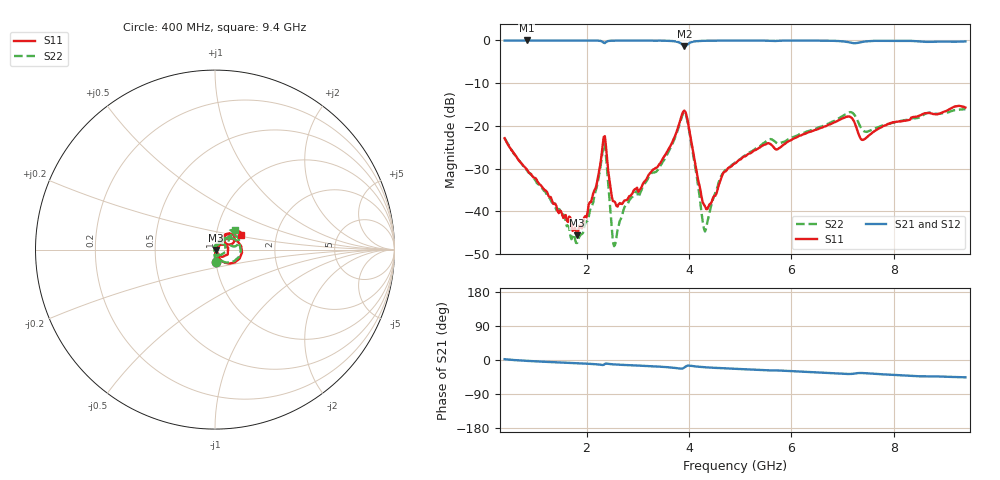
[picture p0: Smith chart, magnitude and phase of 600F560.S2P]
!  American Technical Ceramics  Date:  11/23/05
!  One Norden Lane
!  Huntington Station,  NY.  11746-2102
!  Tel:  (631) 622-4700  Fax:  (631) 622-4748
!  Part Number  600F560  Mounting Orientation: Horizontal
!  Description: Ultra Low ESR Microwave capacitors
!  Application: Coupling, Bypass, Tuning, DC Block
!  Filters, Matching
# GHZ S DB R 50
! Freq  |S11|  S11 Ph  |S21|  S21 Ph  |S12|  S12 Ph  |S22|  S22 Ph
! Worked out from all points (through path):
!   401 points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, 400 MHz to 9.4 GHz, reference 50 ohm
!   highest |S21| = 0.00 dB at 828 MHz (marker M1); lowest = -1.3 dB at 3.91 GHz (marker M2)
!   group delay of S21, straight-line fit = 14.1 ps
!   lowest |S11| = -45.6 dB at 1.818 GHz (marker M3), VSWR 1.01, Z = 50.5 - j0.172 ohm
!   |S11| at or under -10 dB: start of sweep to end of sweep
!   |S22| runs from -48.1 to -16.1 dB; largest |S21 - S12| = 0.0045
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0.4  -22.87 -86.8  -0.02 2.2  -0.03 2.2  -22.88 -87.6
0.828  -30.07 -87.9  0.00 -2.2  -0.02 -2.2  -30.23 -93.3
1.818  -45.56 -18.9  -0.01 -8.6  -0.02 -8.6  -47.37 179.0
1.908  -43.97 9.3  -0.01 -9.1  -0.02 -9.1  -45.29 137.7
2.178  -34.57 41.4  -0.02 -11.1  -0.04 -11.1  -35.20 95.1
2.335  -22.58 9.2  -0.54 -12.8  -0.55 -12.7  -24.12 25.2
2.38  -24.83 -45.1  -0.38 -9.5  -0.40 -9.4  -27.00 -42.0
2.515  -37.57 -34.1  -0.05 -11.4  -0.06 -11.4  -47.01 -140.2
2.56  -37.92 -24.2  -0.04 -11.8  -0.05 -11.8  -47.72 155.4
2.785  -37.34 19.0  -0.04 -13.4  -0.06 -13.3  -38.43 103.7
3.415  -29.06 54.0  -0.04 -17.5  -0.06 -17.5  -29.83 68.0
3.91  -16.40 -6.2  -1.33 -19.9  -1.34 -19.9  -16.82 -2.7
4  -20.48 -51.6  -0.68 -14.9  -0.70 -14.9  -20.80 -51.2
4.315  -38.84 -16.1  -0.08 -19.1  -0.09 -19.1  -44.70 -2.5
4.63  -32.25 62.7  -0.05 -21.4  -0.06 -21.4  -31.65 61.5
4.9  -28.77 59.1  -0.01 -23.2  -0.03 -23.2  -28.57 56.0
5.553  -24.02 53.0  -0.09 -27.4  -0.10 -27.3  -23.21 46.6
6.408  -21.19 59.2  -0.04 -31.9  -0.05 -31.8  -20.89 45.0
7.15  -17.86 32.1  -0.49 -36.9  -0.51 -36.8  -16.76 25.7
7.398  -23.27 36.3  -0.32 -34.5  -0.33 -34.5  -21.02 16.5
7.915  -19.42 52.0  -0.08 -38.7  -0.10 -38.7  -19.49 38.5
9.4  -15.68 29.6  -0.22 -45.6  -0.24 -45.7  -16.08 43.4
